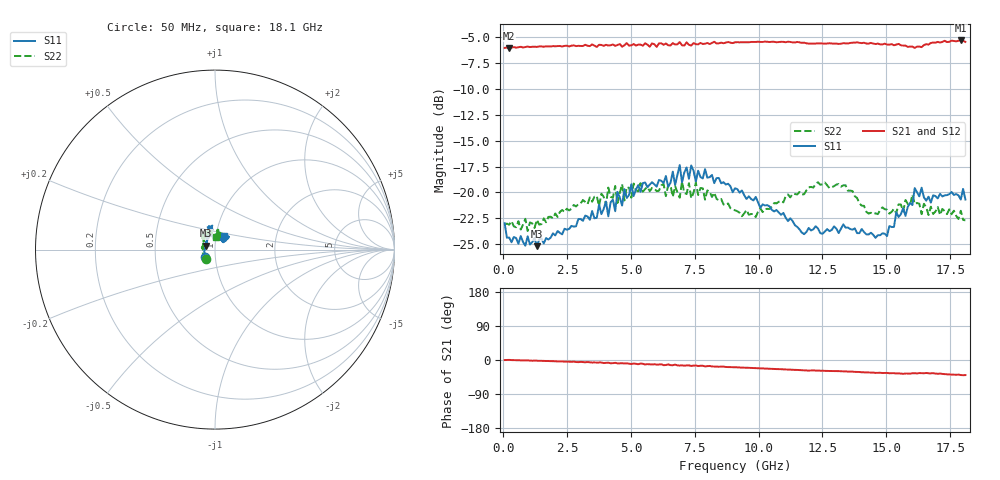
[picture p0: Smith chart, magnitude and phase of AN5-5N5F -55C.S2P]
! Network Analyzer HP8720D.06.14 Serial No. US36140669
!  5 Jul 2005  07:52:28
! Frequency  S11  S21  S12  S22
# HZ  S  DB R 50
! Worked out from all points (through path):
!   201 points, 50 MHz to 18.1 GHz, reference 50 ohm
!   highest |S21| = -5.36 dB at 17.92 GHz (marker M1); lowest = -6.1 dB at 230.5 MHz (marker M2)
!   group delay of S21, straight-line fit = 6.43 ps
!   lowest |S11| = -25.2 dB at 1.313 GHz (marker M3), VSWR 1.12, Z = 45.1 + j1.94 ohm
!   |S11| at or under -10 dB: start of sweep to end of sweep
!   |S22| runs from -23.7 to -19.0 dB; largest |S21 - S12| = 0.017
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5e7  -22.95 -141.9  -6.07 -0.2  -6.04 -0.0  -23.05 -133.4
2.305e8  -24.34 -171.4  -6.09 0.3  -6.09 0.2  -23.10 -174.9
1.3135e9  -25.17 157.2  -5.98 -1.8  -5.94 -1.9  -22.64 156.2
3.1185e9  -22.74 126.4  -5.89 -5.5  -5.90 -5.8  -20.72 138.8
6.09675e9  -18.80 104.3  -5.64 -12.0  -5.60 -11.9  -19.83 117.7
6.7285e9  -19.27 106.6  -5.75 -12.2  -5.88 -13.3  -19.38 110.9
6.909e9  -17.35 104.3  -5.51 -14.8  -5.69 -14.0  -20.50 107.6
6.99925e9  -19.03 103.0  -5.83 -14.0  -5.82 -15.3  -18.95 109.0
7.27e9  -18.68 101.5  -5.77 -14.2  -5.76 -15.7  -19.11 108.2
7.36025e9  -17.40 96.3  -5.85 -15.6  -5.74 -14.5  -20.56 112.5
7.54075e9  -18.96 97.1  -5.72 -14.3  -5.56 -15.9  -19.05 111.9
7.90175e9  -17.75 103.6  -5.67 -16.8  -5.67 -15.8  -20.69 105.0
9.075e9  -19.60 109.8  -5.54 -19.1  -5.53 -19.1  -21.72 96.0
9.88725e9  -20.43 107.2  -5.50 -21.5  -5.47 -21.4  -22.37 82.6
1.21435e10  -23.55 94.1  -5.66 -27.3  -5.62 -27.5  -19.53 81.1
1.3407e10  -23.38 71.5  -5.63 -30.0  -5.60 -30.2  -19.30 82.0
1.43095e10  -24.05 50.0  -5.65 -32.9  -5.62 -33.2  -22.04 87.6
1.512175e10  -23.23 43.0  -5.75 -34.9  -5.65 -34.7  -22.04 82.9
1.57535e10  -22.26 44.6  -5.85 -35.6  -6.02 -36.6  -20.72 72.3
1.61145e10  -19.58 44.7  -6.07 -35.0  -5.87 -35.3  -21.11 68.2
1.79195e10  -20.68 57.8  -5.36 -39.7  -5.24 -39.7  -21.76 87.8
1.81e10  -20.68 57.6  -5.49 -39.8  -5.57 -40.7  -22.69 83.8
